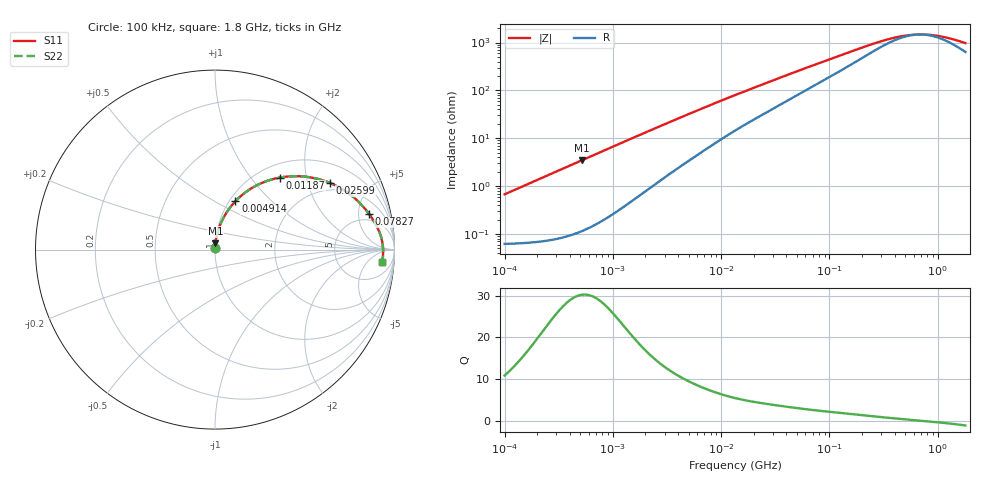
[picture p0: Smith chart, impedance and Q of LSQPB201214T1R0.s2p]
! LSQPB201214T1R0  S-PARAMETER MODEL  ( General Type )
! Model Generated by TAIYO YUDEN Corporation (http://www.ty-top.com)
! Version 1.0
! TAIYO YUDEN Control No. 100901NG22SB-FKC
! Copyright(c) 2010 TAIYO YUDEN CO.,LTD. All Rights Reserved.
! Product Description (link to TY-COMPAS)
! https://ds.yuden.co.jp/TYCOMPAS/or/detail?pn=LSQPB201214T1R0M&u=M
! Products Name : Inductors
! Characteristics :
!  Inductance : 1.0 uH , SRF(min) : 490 MHz , DC Resistance(max) : 0.078 Ohm
!  Rated Current : Saturation :1500 mA , Temp Rise : 1400 mA (40 degC)
!  Case Size : 2.0 x 1.25 / 0.079 x 0.049 [mm/inch] , Thickness : 1.4 / 0.056 [mm/inch]
!  (Conditions: Temperature = 25 degC , DC Bias Current/Voltage = 0A / 0V)
! External Node Assignments :
!  1  o---GGG---o  2
! GND o---------o GND
! Frequency Range : 0.1MHz  -  1800MHz  [ 402 STEP ]
# MHz S RI R 50
! Freq[MHz].  S11 Real  S11 Imag  S21 Real  S21 Imag  S12 Real  S12 Imag  S22 Real  S22 Imag
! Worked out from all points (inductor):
!   401 points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, 100 kHz to 1.8 GHz, reference 50 ohm
!   read as one part in series: L = 1.07 uH near 105 kHz
!   highest Q = 30.2 at 516.1 kHz (marker M1), where L = 1.07 uH
!   self-resonance near 677.1 MHz
!   S11 on the Smith chart (normalised r, x): 100 kHz: 1.00, +0.01; 4.914 MHz: 1.07, +0.63; 11.87 MHz: 1.24, +1.41; 25.99 MHz: 1.69, +2.77; 78.27 MHz: 3.79, +6.72; 1.8 GHz: 14, -15
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0.1  0.000665 0.00671  0.9993 -0.00671  0.9993 -0.00671  0.000665 0.00671
0.516129  0.00234 0.0345  0.9977 -0.0345  0.9977 -0.0345  0.00234 0.0345
1.246616  0.0104 0.0821  0.9896 -0.0821  0.9896 -0.0821  0.0104 0.0821
2.66389  0.0409 0.1655  0.9591 -0.1655  0.9591 -0.1655  0.0409 0.1655
3.662795  0.0705 0.2159  0.9295 -0.2159  0.9295 -0.2159  0.0705 0.2159
4.914404  0.1133 0.2689  0.8867 -0.2689  0.8867 -0.2689  0.1133 0.2689
7.452807  0.2081 0.3446  0.7919 -0.3446  0.7919 -0.3446  0.2081 0.3446
11.86985  0.3604 0.4012  0.6396 -0.4012  0.6396 -0.4012  0.3604 0.4012
13.41641  0.4054 0.4073  0.5946 -0.4073  0.5946 -0.4073  0.4054 0.4073
18.44729  0.523 0.4037  0.477 -0.4037  0.477 -0.4037  0.523 0.4037
25.99364  0.6393 0.372  0.3607 -0.372  0.3607 -0.372  0.6393 0.372
41.39926  0.7616 0.3003  0.2384 -0.3003  0.2384 -0.3003  0.7616 0.3003
69.24595  0.8455 0.2155  0.1545 -0.2155  0.1545 -0.2155  0.8455 0.2155
78.26819  0.8594 0.1972  0.1406 -0.1972  0.1406 -0.1972  0.8594 0.1972
155.4012  0.9101 0.1115  0.0899 -0.1115  0.0899 -0.1115  0.9101 0.1115
253.6402  0.9267 0.0657  0.0733 -0.0657  0.0733 -0.0657  0.9267 0.0657
357.3983  0.9325 0.04  0.0675 -0.04  0.0675 -0.04  0.9325 0.04
542.0029  0.9359 0.0133  0.0641 -0.0133  0.0641 -0.0133  0.9359 0.0133
659.3364  0.9365 0.00158  0.0635 -0.00158  0.0635 -0.00158  0.9365 0.00158
782.6622  0.9367 -0.00866  0.0633 0.00866  0.0633 0.00866  0.9367 -0.00866
1130.179  0.9361 -0.0319  0.0639 0.0319  0.0639 0.0319  0.9361 -0.0319
1800  0.9324 -0.0678  0.0676 0.0678  0.0676 0.0678  0.9324 -0.0678
